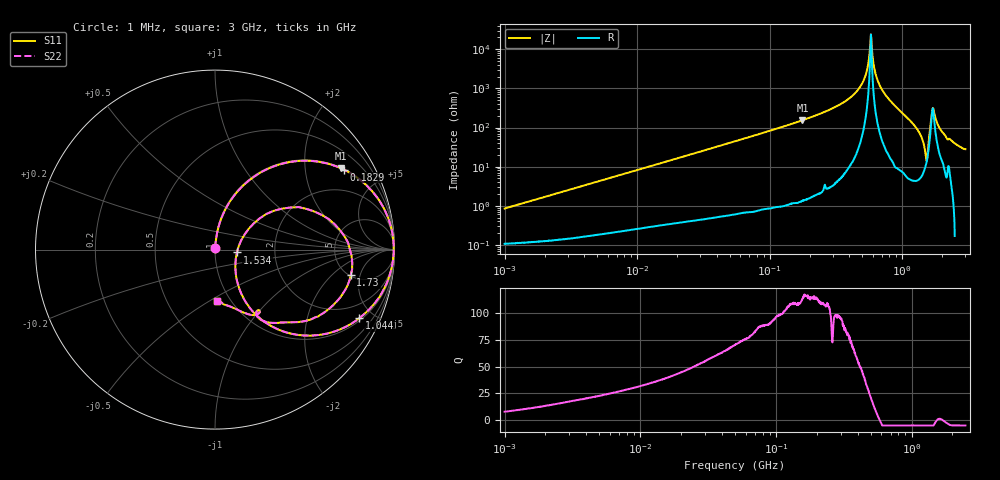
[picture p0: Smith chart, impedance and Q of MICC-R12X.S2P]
!s-Parameter Generated by FASTRON Sdn. Bhd.
!FASTRON P/N : MICC-R12X
!Keysight Technologies,E4991B,MY54100416,A.01.15
!Date: Wed Aug 26 15:41:14 2026
!Version  : Rev00 Wed Aug 26 15:41:14 2026
!Data & Calibration Information:
!PortZ  Port1:50+j0  Port2:50+j0
!When reading, reference impedance value at option line is always used.
! Remarks : This data is being provided solely for informational purposes.
!Freq	S11	S21	S12	S22
# Hz S dB R 50
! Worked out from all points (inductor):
!   1601 points, 1 MHz to 3 GHz, reference 50 ohm
!   read as one part in series: L = 134 nH near 1.041 MHz
!   highest Q = 116 at 176.6 MHz (marker M1), where L = 138 nH
!   self-resonance near 581.2 MHz
!   S11 on the Smith chart (normalised r, x): 1 MHz: 1.00, +0.02; 182.9 MHz: 1.03, +3.20; 1.044 GHz: 1.13, -4.15; 1.534 GHz: 1.28, -0.04; 1.73 GHz: 5.13, -3.57; 3 GHz: 0.87, -0.54
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1000000  -41.40 82.3  -0.01 -0.5  -0.01 -0.5  -41.40 82.3
3804036  -30.00 85.3  -0.02 -1.8  -0.02 -1.8  -30.00 85.3
1.447069e7  -18.65 81.8  -0.09 -6.7  -0.09 -6.7  -18.65 81.8
5.477226e7  -7.87 65.4  -0.83 -23.8  -0.83 -23.8  -7.87 65.4
1.766402e8  -1.57 32.9  -5.29 -56.6  -5.29 -56.6  -1.57 32.9
1.829372e8  -1.47 31.9  -5.55 -57.6  -5.55 -57.6  -1.47 31.9
2.083556e8  -1.12 28.0  -6.58 -61.5  -6.58 -61.5  -1.12 28.0
3.334925e8  -0.32 14.8  -11.83 -74.4  -11.83 -74.4  -0.32 14.8
4.480278e8  -0.09 7.1  -18.13 -81.5  -18.13 -81.5  -0.09 7.1
5.205962e8  -0.04 3.1  -25.31 -83.0  -25.31 -83.0  -0.04 3.1
5.81181e8  -0.04 0.0  -47.60 -2.5  -47.60 -2.5  -0.04 0.0
6.553423e8  -0.06 -3.7  -23.87 82.0  -23.87 82.0  -0.06 -3.7
7.925923e8  -0.21 -10.5  -14.75 77.4  -14.75 77.4  -0.21 -10.5
1.0437e9  -1.01 -25.4  -7.35 62.8  -7.35 62.8  -1.01 -25.4
1.340405e9  -4.59 -50.4  -2.24 36.0  -2.24 36.0  -4.59 -50.4
1.437675e9  -8.42 -59.2  -1.22 22.0  -1.22 22.0  -8.42 -59.2
1.534307e9  -18.18 -7.2  -1.13 1.0  -1.13 1.0  -18.18 -7.2
1.621129e9  -5.65 27.0  -4.66 -23.9  -4.66 -23.9  -5.65 27.0
1.730092e9  -2.27 -10.6  -11.00 30.2  -11.00 30.2  -2.27 -10.6
1.818868e9  -2.95 -28.0  -6.02 42.0  -6.02 42.0  -2.95 -28.0
1.950859e9  -4.43 -42.4  -3.25 36.0  -3.25 36.0  -4.43 -42.4
3e9  -10.84 -87.4  0.24 16.2  0.24 16.2  -10.84 -87.4
